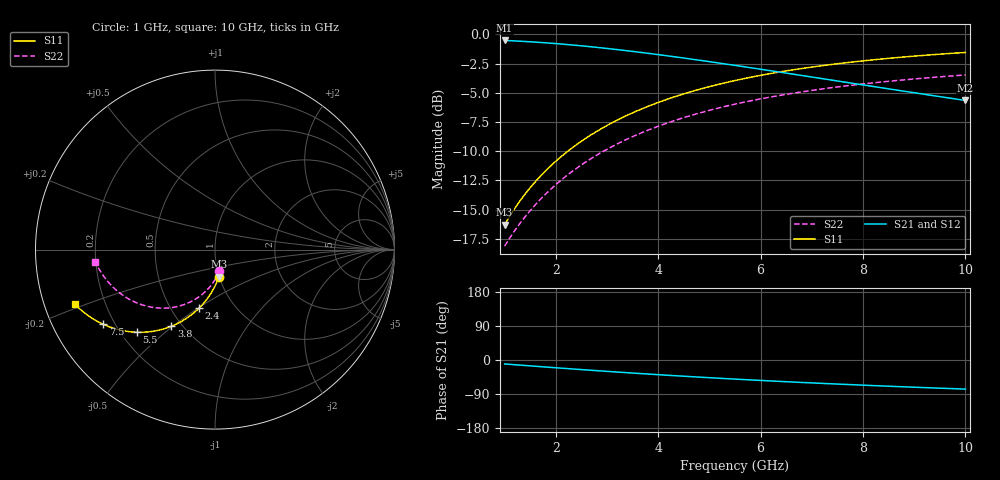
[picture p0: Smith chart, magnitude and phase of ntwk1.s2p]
! Created Thu Nov 11 11:09:06 2010
# ghz S ri R 50
! 2 Port Network Data from SP1.SP block
! freq  reS11  imS11  reS21  imS21  reS12  imS12  reS22  imS22
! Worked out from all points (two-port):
!   91 points, 1 GHz to 10 GHz, reference 50 ohm
!   highest |S21| = -0.52 dB at 1 GHz (marker M1); lowest = -5.7 dB at 10 GHz (marker M2)
!   |S21| within 3 dB of the highest: start of sweep to 6.804 GHz
!   lowest |S11| = -16.3 dB at 1 GHz (marker M3), VSWR 1.36, Z = 49.8 - j15.5 ohm
!   |S11| at or under -10 dB: start of sweep to 2.236 GHz
!   |S22| runs from -18.1 to -3.5 dB; largest |S21 - S12| = 0
!   S11 on the Smith chart (normalised r, x): 1 GHz: 1.00, -0.31; 2.4 GHz: 0.69, -0.50; 3.8 GHz: 0.44, -0.49; 5.5 GHz: 0.26, -0.40; 7.5 GHz: 0.16, -0.30; 10 GHz: 0.09, -0.19
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1  0.0218 -0.1515  0.9267 -0.1701  0.9267 -0.1701  0.0235 -0.1217
1.1  0.0165 -0.1658  0.9215 -0.1863  0.9215 -0.1863  0.0185 -0.1331
1.3  0.00459 -0.1937  0.9097 -0.2179  0.9097 -0.2179  0.00742 -0.1551
1.6  -0.0164 -0.2335  0.8888 -0.2633  0.8888 -0.2633  -0.0122 -0.1861
1.8  -0.0323 -0.2584  0.873 -0.2921  0.873 -0.2921  -0.027 -0.2053
2  -0.0496 -0.2821  0.8558 -0.3195  0.8558 -0.3195  -0.0431 -0.2233
2.4  -0.0877 -0.325  0.8179 -0.3702  0.8179 -0.3702  -0.0784 -0.255
2.5  -0.0979 -0.3349  0.8078 -0.3819  0.8078 -0.3819  -0.0878 -0.262
2.8  -0.1296 -0.362  0.7763 -0.4149  0.7763 -0.4149  -0.1172 -0.2808
3.1  -0.1629 -0.3856  0.7432 -0.4443  0.7432 -0.4443  -0.1478 -0.2963
3.4  -0.1971 -0.4057  0.7091 -0.4704  0.7091 -0.4704  -0.1792 -0.3085
3.8  -0.2437 -0.4273  0.6627 -0.5  0.6627 -0.5  -0.2218 -0.3197
4  -0.2671 -0.4359  0.6393 -0.5126  0.6393 -0.5126  -0.2431 -0.3232
4.7  -0.3483 -0.4555  0.5582 -0.5464  0.5582 -0.5464  -0.3163 -0.3254
5.1  -0.3933 -0.4601  0.5132 -0.5592  0.5132 -0.5592  -0.3564 -0.3204
5.5  -0.4367 -0.4604  0.4696 -0.5678  0.4696 -0.5678  -0.3947 -0.3114
6.2  -0.508 -0.4524  0.3979 -0.5745  0.3979 -0.5745  -0.4565 -0.2878
7  -0.5813 -0.4327  0.3238 -0.5716  0.3238 -0.5716  -0.5183 -0.251
7.5  -0.6226 -0.4161  0.2818 -0.5656  0.2818 -0.5656  -0.5519 -0.2241
8.5  -0.6947 -0.3758  0.2079 -0.5466  0.2079 -0.5466  -0.6081 -0.1644
9.2  -0.7376 -0.3438  0.1634 -0.5295  0.1634 -0.5295  -0.6392 -0.1196
10  -0.7796 -0.3049  0.1192 -0.5077  0.1192 -0.5077  -0.6672 -0.067
